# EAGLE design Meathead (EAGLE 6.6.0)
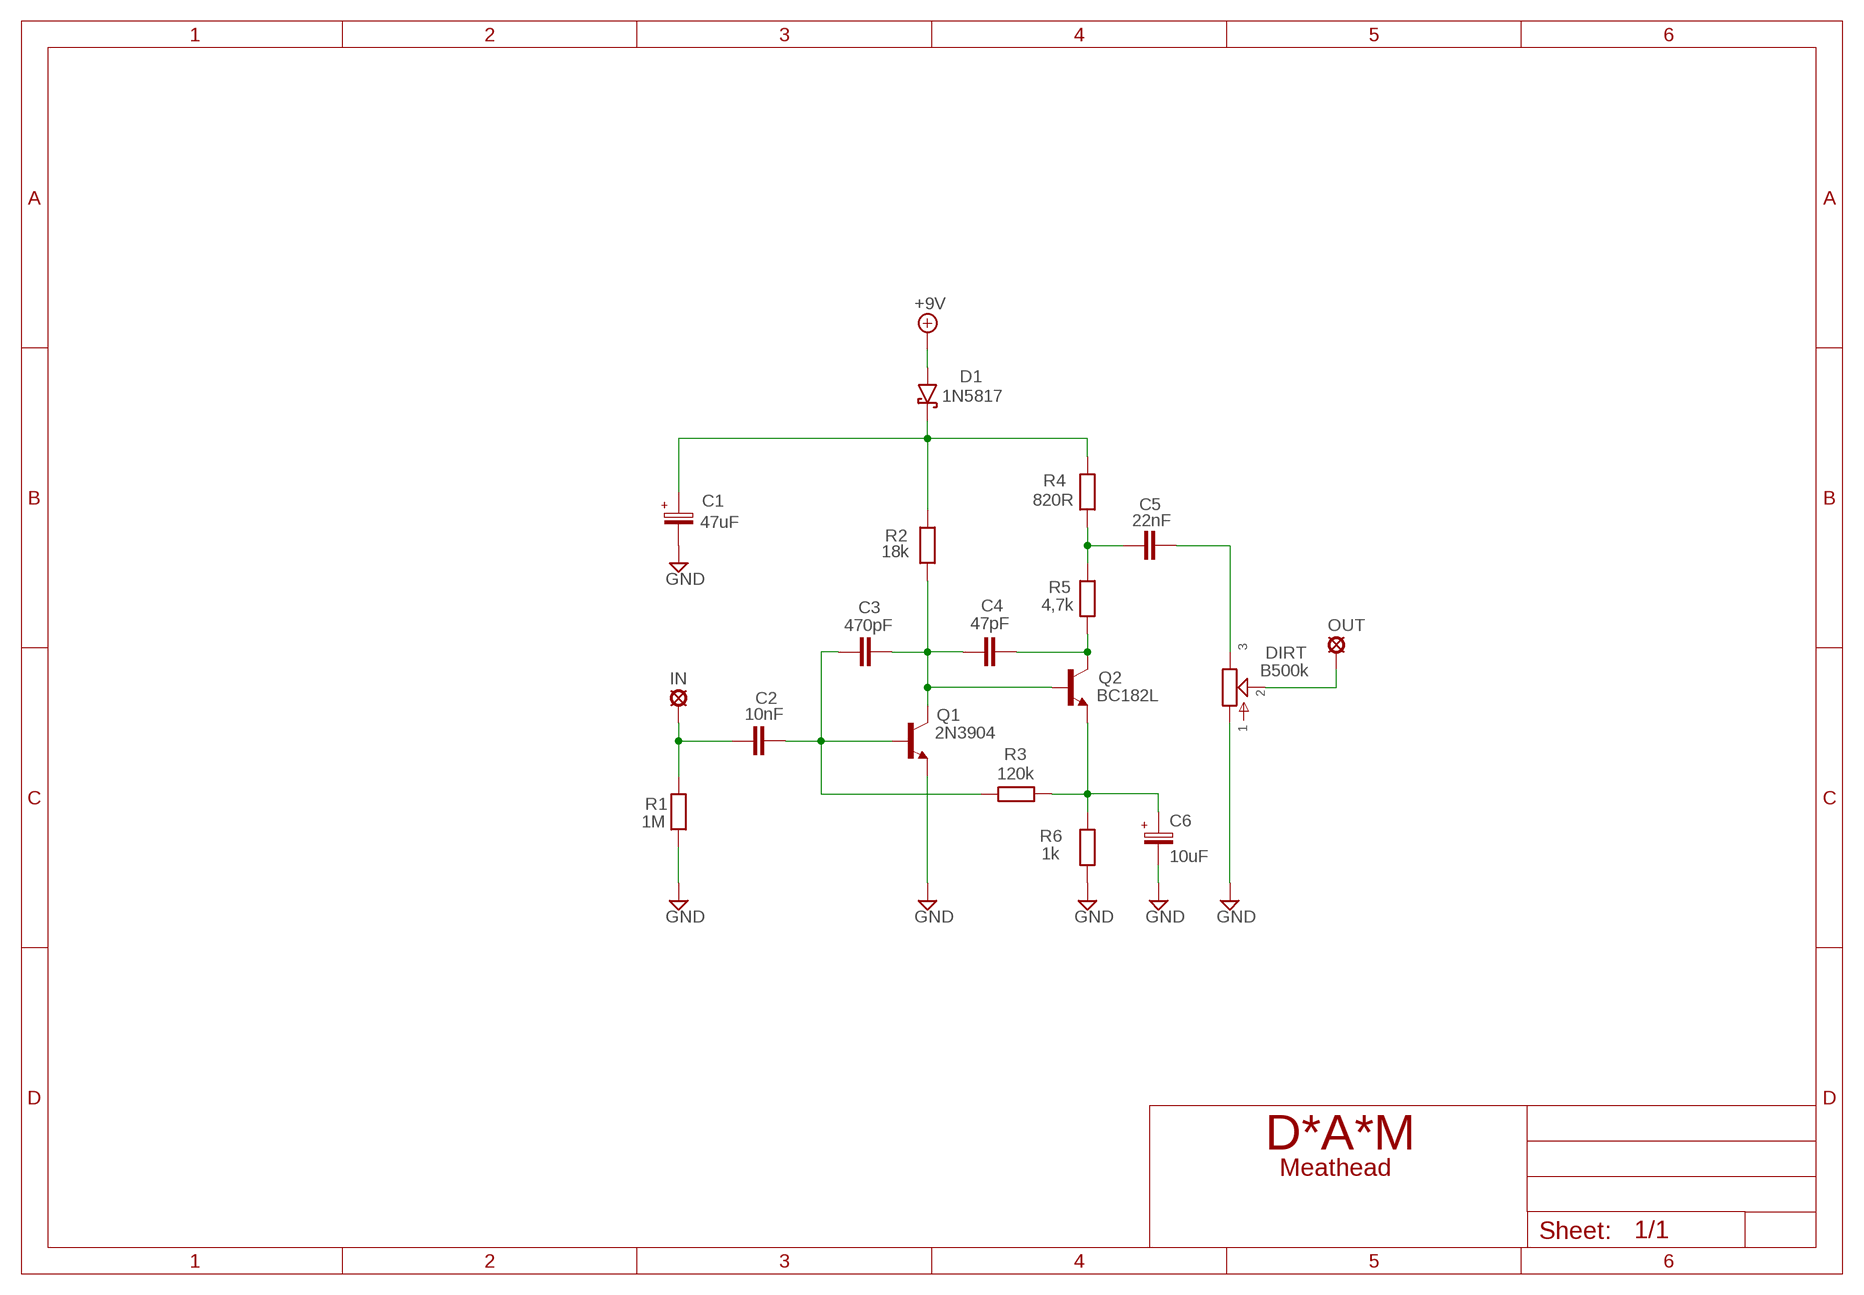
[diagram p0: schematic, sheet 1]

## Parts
+9V  +9V  +9V(T)1  [ROUND]
C1  47uF  063-EU  [063_025]
C2  10nF  1NF-15NF  [3,5MM]
C3  470pF  050X030_0251  [050X030_025]
C4  47pF  050X030_0251  [050X030_025]
C5  22nF  22NF-82NF"  [4,5MM]
C6  10uF  063-EU  [063_025]
D1  1N5817  [DO41-3]
DIRT  B500k  POT-EU16MM  [16MM]
GND  GND  GND(T)1  [ROUND]
GND4  GND  GND(T)1  [ROUND]
IN  MCS10B  [MCS10B]
OUT  MCS10B  [MCS10B]
Q1  2N3904  [TO92-]
Q2  BC182L  [TO92-BCE]
R1  1M  6MM-EU3  [R0207/3]
R2  18k  6MM-EU3  [R0207/3]
R3  120k  6MM-EU3  [R0207/3]
R4  820R  6MM-EU3  [R0207/3]
R5  4,7k  6MM-EU3  [R0207/3]
R6  1k  6MM-EU3  [R0207/3]

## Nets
+9V: +9V.1(+9V) D1.A
GND: C1.- C6.- DIRT.1 GND4.1(GND) GND.1(GND) Q1.3(E) R1.1 R6.1
N$1: C2.1 IN.MP R1.2
N$2: C1.+ D1.C R2.2 R4.2
N$3: C5.1 R4.1 R5.2
N$4: C4.2 Q2.C R5.1
N$5: C5.2 DIRT.3
N$6: DIRT.2 OUT.MP
N$7: C6.+ Q2.E R3.1 R6.2
N$8: C3.2 C4.1 Q1.1(C) Q2.B R2.1
N$9: C2.2 C3.1 Q1.2(B) R3.2

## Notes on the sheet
- D*A*M

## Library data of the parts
+9V = gm-supply:+9V(T): +9V Voltage Supply
C1 C6 = Elektrolyytit:063-EU
C2 = Mylar Kondensaattorit:1NF-15NF: 1nF-15nF
C3 C4 = Keraamiset kondensaattorit:050X030_025: 47 - 120pF
C5 = Mylar Kondensaattorit:22NF-82NF: 22nF-82nF
D1 = Diodit:1N5817
DIRT = gm-pots:POT-EU
GND GND4 = gm-supply:GND(T): Ground
IN OUT = Padit:MCS10B: SOLDER PAD
Q1 = Transistorit:2N3904: NPN Transistor
Q2 = Transistorit:BC182L: BC182L Top Boost Unit transistor.
R1-R6 = Vastukset:6MM-EU: 6mm Resistors (European schematic symbol)

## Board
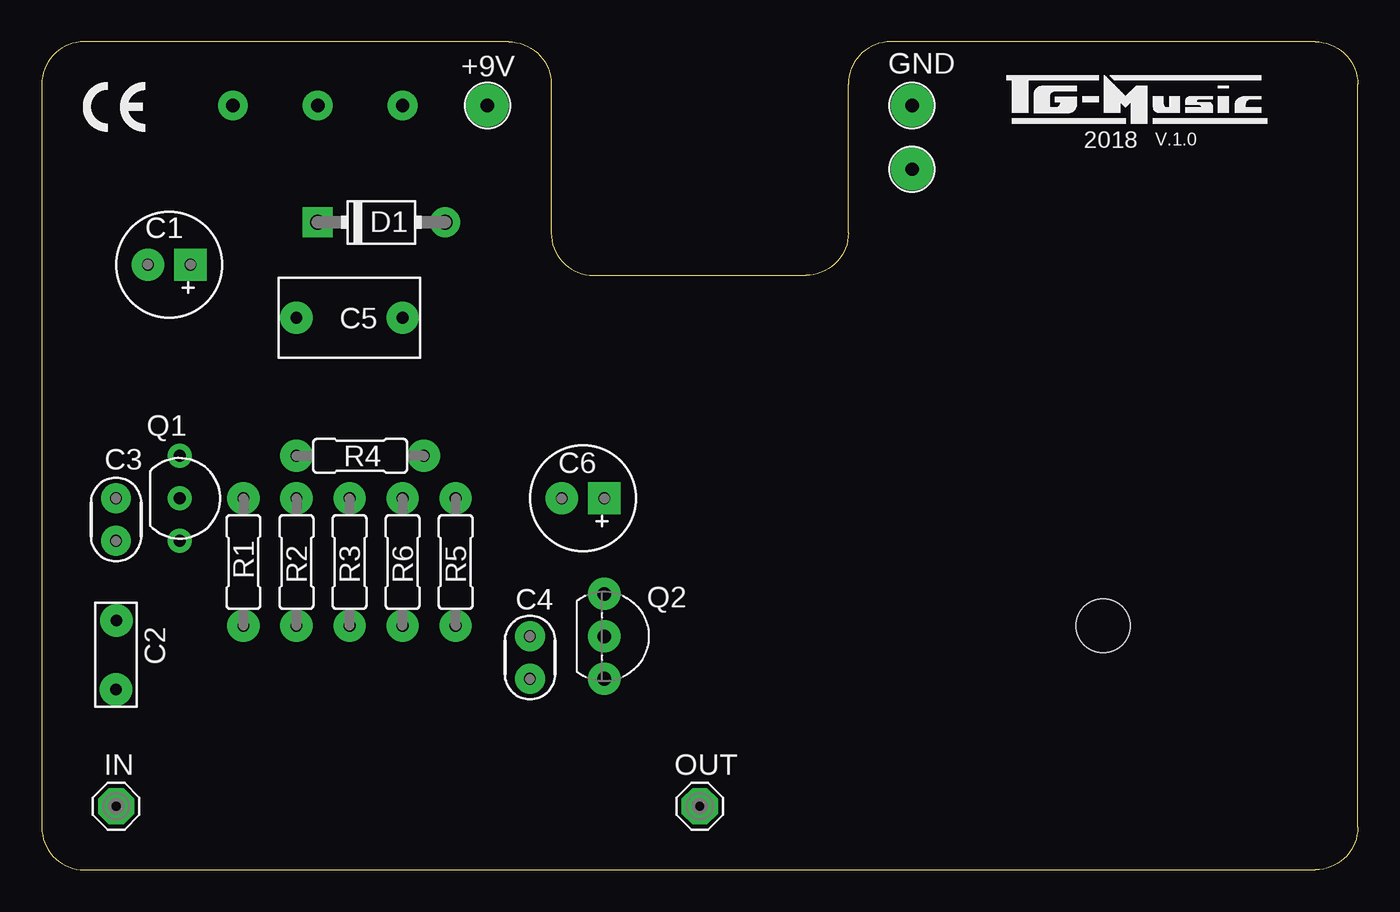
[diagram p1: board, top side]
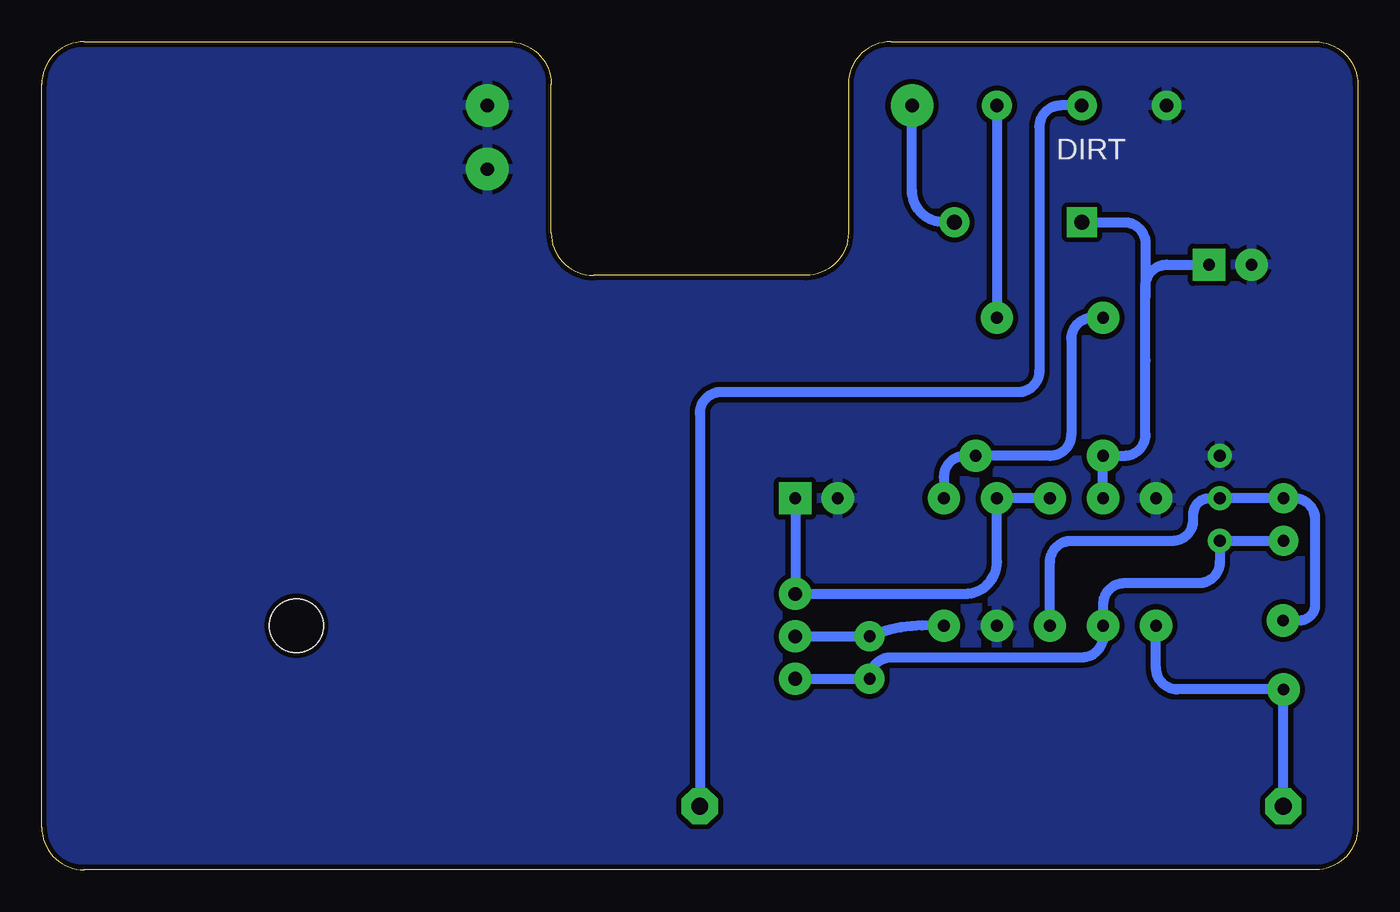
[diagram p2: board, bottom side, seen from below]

Size 78.74 x 49.53 mm. Coordinates in mm from the lower left corner, seen from the top.
Outline: 7.62,49.53 3.81,49.53
Outline: 78.74,2.54 78.74,46.99 arc90 76.2,49.53 50.8,49.53 arc90 48.26,46.99 48.26,38.1 arc-90 45.72,35.56 33.02,35.56 arc-90 30.48,38.1 30.48,46.99 arc90 27.94,49.53 2.54,49.53 arc90 0,46.99 0,2.54 arc90 2.54,0 76.2,0 arc90 78.74,2.54
Copper layers (1*16): Top 0.035mm / dielectric 1.5mm / Bottom 0.035mm
Design rules "ITEADstudio": minimum track width 10mil, minimum drill 12mil, track to track 12mil, track to pad 12mil, pad to pad 12mil, via to via 12mil, smd to smd 0mil, copper to edge 12mil, drill to drill 12mil, minimum pad ring 10mil, minimum via ring 6mil, stop-mask expansion 4mil, vias tented up to drill 100mil, thermal gap 10mil
Holes 3.2 mm at 63.5,14.61

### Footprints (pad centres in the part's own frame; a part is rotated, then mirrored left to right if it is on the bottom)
ROUND = drill 0.8 pad 2.54: 1 0,0
063_025 = drill 0.7 pad 1.93 square: + -1.27,0 | drill 0.7 pad 1.93: - 1.27,0
3,5MM = drill 0.7 pad 1.93: 1 -1.905,0; 2 2.221,-0.016
050X030_025 = drill 0.7 pad 1.778: 1 -1.27,0; 2 1.27,0
4,5MM = drill 0.7 pad 1.93: 1 -3.175,0; 2 3.175,0
DO41-3 = drill 0.9 pad 1.778: A 3.81,0 | drill 0.9 pad 1.778 square: C -3.81,0
16MM = drill 0.8 pad 1.778: 1 5.08,0; 2 0,0; 3 -5.08,0
MCS10B = drill 1.016 pad 2.159 octagon: MP 0,0
TO92- = drill 0.7 pad 1.422: 1 2.54,0; 2 0,0; 3 -2.54,0
TO92-BCE = drill 0.813 pad 1.93: B 2.54,0; C 0,0; E -2.54,0
R0207/3 = drill 0.7 pad 1.93: 1 -3.81,0; 2 3.81,0

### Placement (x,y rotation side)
+9V  26.67,45.72 0 top
C1  7.62,36.2 180 top
C2  4.45,12.7 90 top
C3  4.45,20.95 270 top
C4  29.21,12.7 90 top
C5  18.41,33.02 0 top
C6  32.38,22.23 180 top
D1  20.32,38.73 0 top
DIRT  16.51,45.72 0 bottom
GND  52.07,45.72 0 top
GND4  52.07,41.91 0 top
IN  4.45,3.81 0 top
OUT  39.37,3.81 0 top
Q1  8.26,22.23 270 top
Q2  33.66,13.97 270 top
R1  12.06,18.41 270 top
R2  15.24,18.41 90 top
R3  18.41,18.41 270 top
R4  19.05,24.77 180 top
R5  24.77,18.41 90 top
R6  21.59,18.41 90 top

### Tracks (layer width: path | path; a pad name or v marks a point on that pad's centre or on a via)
+9V
  Bottom 0.61: +9V.1 26.67,40.64 arc-90 24.77,38.73 D1.A
GND
  pour Bottom: 0,1.27 0,46.99 arc-90 2.54,49.53 27.94,49.53 arc-90 30.48,46.99 30.48,38.1 arc90 33.02,35.56 45.72,35.56 arc90 48.26,38.1 48.26,47.62 arc-90 50.16,49.53 76.2,49.53 arc-90 78.74,46.99 78.74,1.91 arc-90 76.83,0 1.27,0 arc-90
N$1
  Bottom 0.61: IN.MP C2.1 10.79,10.79 arc90 12.06,12.06 R1.2
N$2
  Bottom 0.61: R2.2 R4.2 13.97,24.77 arc-90 12.7,26.04 12.7,30.48 12.7,34.29 | 12.7,34.29 12.7,34.92 arc90 11.43,36.2 C1.+ | D1.C 13.97,38.73 arc90 12.7,37.47 12.7,34.29
N$3
  Bottom 0.61: R5.2 24.77,23.5 arc90 23.5,24.77 R4.1 18.41,24.77 arc-90 17.14,26.04 17.14,31.75 arc90 15.88,33.02 C5.1
N$4
  Bottom 0.61: Q2.C C4.2 arc25 25.4,14.61 R5.1
N$5
  Bottom 0.61: DIRT.3 C5.2
N$6
  Bottom 0.61: DIRT.2 17.78,45.72 arc-90 19.05,44.45 19.05,29.84 arc90 20.32,28.57 38.1,28.57 arc-90 39.37,27.3 OUT.MP
N$7
  Bottom 0.61: C6.+ Q2.E 23.5,16.51 arc-90 21.59,18.41 R6.2 R3.1
N$8
  Bottom 0.61: Q2.B C4.1 arc90 27.94,12.7 16.51,12.7 arc-90 15.24,13.97 R2.1 15.24,15.88 arc90 13.97,17.14 9.53,17.14 arc-90 8.26,18.41 Q1.1 C3.2
N$9
  Bottom 0.61: C2.2 3.49,14.92 arc-90 2.54,15.88 2.54,20.95 arc-90 3.81,22.23 C3.1 Q1.2 8.89,22.23 arc-90 9.84,21.28 9.84,20.92 arc90 11.08,19.68 17.14,19.68 arc-90 18.41,18.41 R3.2 18.28,14.61

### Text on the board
tNames: 2018 | V.1.0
